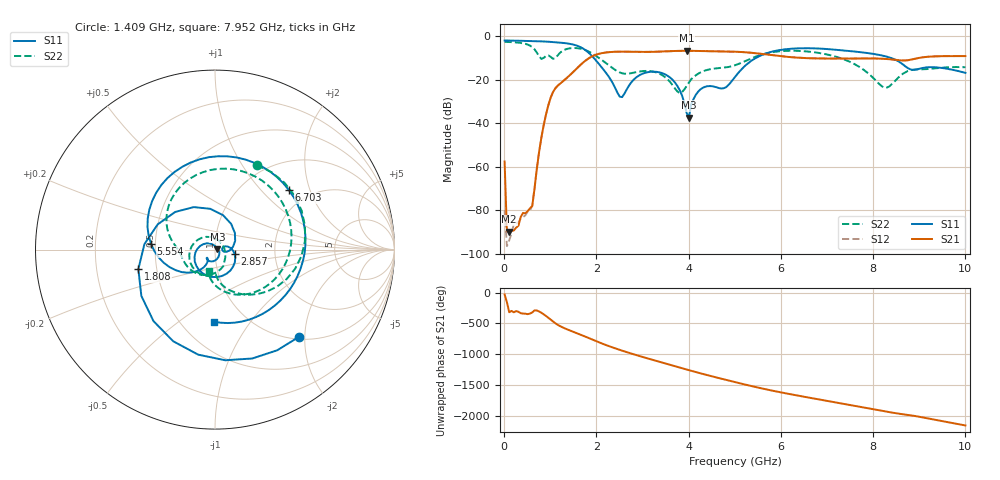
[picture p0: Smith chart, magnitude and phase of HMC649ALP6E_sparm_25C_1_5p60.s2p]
!Analog Devices Inc..
!GaAs MMIC 6-BIT DIGITAL PHASE SHIFTER, 3 - 6 GHz
!Filename: HMC649ALP6E_sparm_25C_1_5p60.s2p
!  :25C = 25degC
!  :_1_ = Sn1
!  :_5p60  = 5.625 state
!Device type:
!2 Port Calibration to sma connectors
!Phase Shifter:  0.000
!	Vss= -5V, Vdd= +5V , control Voltage = 0/ +5V
!Freq	S11	S11	S21	S21	S12	S12	S22	S22
! GHz	Mag dB	Degrees	Mag dB	Degrees	Mag dB	Degrees	Mag dB	Degrees
# GHZ S DB R 50.0
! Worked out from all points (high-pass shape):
!   201 points, 10 MHz to 10 GHz, reference 50 ohm
!   highest |S21| = -6.66 dB at 3.956 GHz (marker M1); lowest = -89.9 dB at 109.9 MHz (marker M2)
!   |S21| within 3 dB of the highest: 1.871 GHz to 6.255 GHz (4.384 GHz wide, 108 % of centre); 9.078 GHz to end of sweep
!   lowest |S11| = -37.4 dB at 4.006 GHz (marker M3), VSWR 1.03, Z = 51.3 + j0.323 ohm
!   |S11| at or under -10 dB: 1.945 GHz to 5.454 GHz (3.509 GHz wide, 94.9 % of centre); 8.391 GHz to end of sweep
!   |S22| runs from -26.1 to -2.6 dB; largest |S21 - S12| = 0.0013
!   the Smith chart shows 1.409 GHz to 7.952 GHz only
!   S11 on the Smith chart (normalised r, x): 1.409 GHz: 1.05, -1.87; 1.808 GHz: 0.39, -0.11; 2.857 GHz: 1.24, -0.06; 5.554 GHz: 0.47, +0.04; 6.703 GHz: 1.58, +1.45; 7.952 GHz: 0.71, -0.68
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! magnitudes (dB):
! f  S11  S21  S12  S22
! 10 MHz  -1.9  -57.6  -79.9  -2.6
! 59.95 MHz  -1.9  -89.7  -96.5  -2.6
! 109.9 MHz  -2.0  -89.9  -93.8  -2.6
! 609.4 MHz  -2.2  -78.1  -77.8  -5.0
! 759.2 MHz  -2.3  -53.0  -53.0  -9.3
! 959 MHz  -2.5  -31.6  -31.6  -8.8
! 1.409 GHz  -3.4  -18.2  -18.2  -5.6
! 1.708 GHz  -5.6  -12.2  -12.1  -6.0
! 1.808 GHz  -7.1  -10.5  -10.5  -6.8
! 2.507 GHz  -27.8  -7.1  -7.1  -16.6
! 2.857 GHz  -19.0  -7.1  -7.1  -16.5
! 3.357 GHz  -16.5  -7.1  -7.0  -17.1
! 3.756 GHz  -22.9  -6.7  -6.7  -25.4
! 3.956 GHz  -35.2  -6.7  -6.7  -22.9
! 4.006 GHz  -37.4  -6.7  -6.7  -21.3
! 4.256 GHz  -24.4  -6.8  -6.8  -16.6
! 5.005 GHz  -18.7  -7.1  -7.1  -13.3
! 5.554 GHz  -8.9  -8.0  -8.0  -8.6
! 6.703 GHz  -5.5  -10.1  -10.1  -7.3
! 7.952 GHz  -7.9  -10.2  -10.2  -18.1
! 8.352 GHz  -9.7  -10.5  -10.5  -23.0
! 10 GHz  -16.8  -9.1  -9.1  -14.2
